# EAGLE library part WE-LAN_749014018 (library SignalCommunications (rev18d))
WE-LAN LAN Transformer 10/100 Base T - Compliant with IEEE 802.3, IEEE 802.3af and IEEE 802.3at standards - SMT -- Ethernet -- Power over Ethernet -- 1 Gigabit Ethernet -- Compliant with most IC's for ethernet applications like Intel, AMD, Globespan and Realtek -- Hub, Router, Switch Details see: http://katalog.we-online.de/en/pbs/WE-LAN/749014018 2016 (C) Würth Elektronik
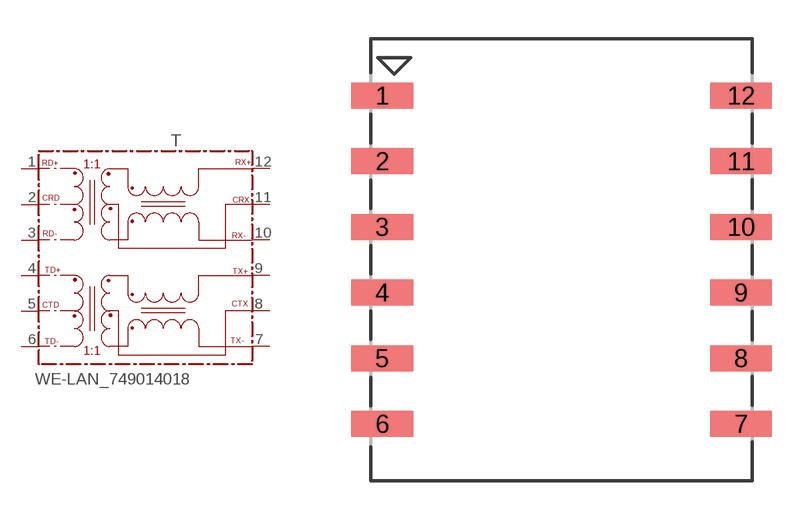
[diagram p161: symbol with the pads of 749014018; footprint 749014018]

Designator prefix T

## WE-LAN_749014018  [749014018]
1  RD+
2  CRD
3  RD-
4  TD+
5  CTD
6  TD-
7  TX-
8  CTX
9  TX+
10  RX-
11  CRX
12  RX+

## Footprint 749014018 (pad centres in mm)
smd 2.39 x 1: 1 -6.935,6.35; 2 -6.935,3.81; 3 -6.935,1.27; 4 -6.935,-1.27; 5 -6.935,-3.81; 6 -6.935,-6.35; 7 6.935,-6.35; 8 6.935,-3.81; 9 6.935,-1.27; 10 6.935,1.27; 11 6.935,3.81; 12 6.935,6.35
